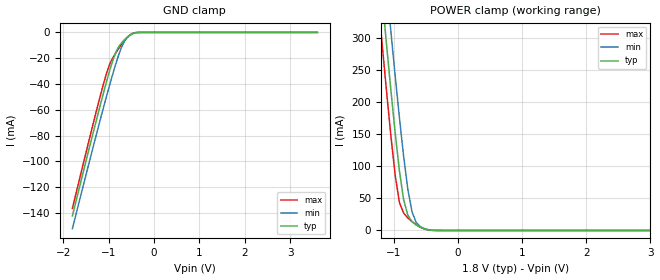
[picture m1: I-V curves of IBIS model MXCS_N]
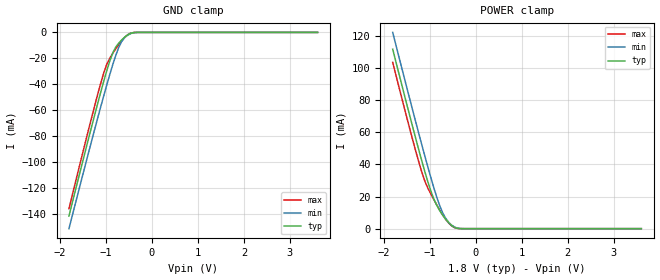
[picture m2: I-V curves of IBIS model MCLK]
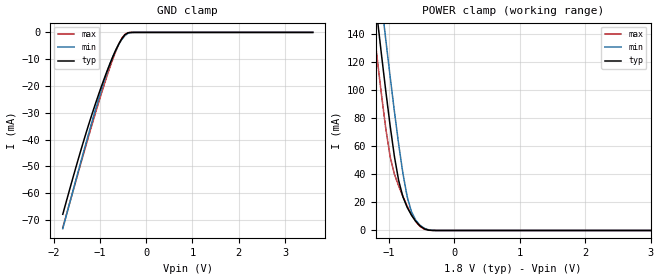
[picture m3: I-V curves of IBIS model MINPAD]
| Created by SiliconSmart  O-2018.09-SP2-3
[IBIS Ver]   4.0
[File Name]   as1101wa_rev1p4.ibs
[File Rev]   1.4
[Date]   Thursday Mar 21 2024
|[Source]   Avalanche Team
|[Notes]   Generated IBIS models from Silicon Smart
|[Rev 1.0]  Initial Release based on extracted netlist
|   Characterization
|[Rev 1.1]  Update Package RLC
|[Rev 1.2]  Recharacterize MIOPAD with Hspice run in high accuracy mode
|[Rev 1.3]  Recharacterize with Hspice to align with datasheet parameter
|[Rev 1.4]  Update the pin to the package pinout assignment
|[Disclaimer]   THE MODEL LIBRARIES ARE PROVIDED AS IS.
|[Copyright]   Copyright 2019, Avalanche Technology., All Rights Reserved
[Component]   AS10xx101_WSON
[Manufacturer] Avalanche Technology
| CONTENT :
| This file contains IBIS MODEL for PSRAM device
| AS1001101 AS1004101 AS1008101 AS1016101
| USAGE :
| The models are derived for the 1.71V to 2.0V I/O Operation.
| Temperatures for model generation: typ: 25, max: -40, min: 105
| Voltages : typ: 1.8V, min: 1.71V, max: 2.0V
| PACKAGES SUPPORTED :
| 8-pad WSON (5.0mm x 6.0mm)
| VERIFICATION :
| Errors  : 0
| Warnings: 10
| All warnings due to non-monotonic data
[Package]
|variable   typ   min   max
R_pkg   8.90E-04   8.89E-04  8.91E-04
L_pkg   1.185E-09  1.18E-09  1.19E-09
C_pkg   2.30E-13   2.21E-13  2.39E-13
[Pin]   signal_name   model_name   R_pin   L_pin   C_pin
1   CS#   MXCS_N   1.05E-01  1.35E-09  9.16E-14
2   SO   MIOPAD   1.05E-01  1.35E-09  9.16E-14
3   WP#   MINPAD   1.05E-01  1.35E-09  9.16E-14
5   SI   MINPAD   3.75E-02  3.89E-10  4.24E-14
6   CLK   MCLK   3.75E-02  3.89E-10  4.24E-14
7   HOLD#   MINPAD   3.75E-02  3.89E-10  4.24E-14
4   VSS   GND   NA   NA   NA
8   VCC   POWER   NA   NA   NA
[Model Selector] MIOPAD
| Model Description
M3_IOPAD_NVCR_OB04   45 Ohms drv strength
| Models and submodels in the file (4): MXCS_N (Input), MCLK (Input), MINPAD (Input), M3_IOPAD_NVCR_OB04 (Output)
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| XCS_N
[Model] MXCS_N
Model_type Input
Enable   Active-High
Vinl  =  0.54
Vinh  =  1.26
| Capacitance  typ   min   max
C_comp   3.084351e-12   2.813138e-12   3.400928e-12
| Variables   typ   min   max
[GND Clamp Reference]   0   0   0
[POWER Clamp Reference]   1.8   1.71   2
[Pulldown Reference]   0   0   0
[Pullup Reference]   1.8   1.71   2
[Temperature Range]   25   105   -40
[Voltage Range]   1.8   1.71   2
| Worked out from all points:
|   GND clamp passes 1 mA (typ) near -0.48 V on its own axis
|   POWER clamp passes 1 mA (typ) near -0.46 V on its own axis
[GND Clamp]
| Voltage   I(typ)   I(min)   I(max)
-1.8V     -142.2mA   -152mA     -136.3mA
-1.303V   -72.38mA   -83.46mA   -65.31mA
-1.173V   -54.66mA   -65.96mA   -47.51mA
-1.043V   -37.59mA   -48.87mA   -31.14mA
-977.6mV  -29.52mA   -40.56mA   -24.56mA
-847.2mV  -15.78mA   -24.8mA    -16.17mA
-716.9mV  -8.18mA    -11.5mA    -9.334mA
-651.7mV  -5.669mA   -6.824mA   -6.326mA
-586.6mV  -3.535mA   -3.869mA   -3.746mA
-456.2mV  -640.4uA   -879uA     -510.8uA
-325.9mV  -14.45uA   -51.53uA   -3.775uA
3.6V      0A         0A         0A
[POWER Clamp]
| Voltage   I(typ)   I(min)   I(max)
-1.8V     1.062A     1.152A     991.6mA
-1.238V   424.5mA    517.2mA    351.4mA
-1.173V   353.2mA    445.8mA    280.1mA
-1.108V   283.2mA    375.4mA    210.6mA
-1.043V   215.2mA    306.4mA    144.3mA
-977.6mV  150.6mA    239.2mA    85.02mA
-912.4mV  92.52mA    174.9mA    43.53mA
-847.2mV  47.97mA    115.2mA    27.04mA
-716.9mV  13.61mA    29.16mA    13.92mA
-651.7mV  8.604mA    12.47mA    8.943mA
-325.9mV  22.75uA    80.1uA     9.962uA
3.6V      0A         0A         0A
| CLK
[Model] MCLK
Model_type Input
Enable   Active-High
Vinl  =  0.54
Vinh  =  1.26
| Capacitance  typ   min   max
C_comp   2.700843e-12   2.498345e-12   2.928788e-12
| Variables   typ   min   max
[GND Clamp Reference]   0   0   0
[POWER Clamp Reference]   1.8   1.71   2
[Pulldown Reference]   0   0   0
[Pullup Reference]   1.8   1.71   2
[Temperature Range]   25   105   -40
[Voltage Range]   1.8   1.71   2
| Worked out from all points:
|   GND clamp passes 1 mA (typ) near -0.48 V on its own axis
|   POWER clamp passes 1 mA (typ) near -0.47 V on its own axis
[GND Clamp]
| Voltage   I(typ)   I(min)   I(max)
-1.8V     -141.2mA   -150.9mA   -135.5mA
-1.303V   -71.9mA    -82.87mA   -64.94mA
-1.173V   -54.3mA    -65.5mA    -47.25mA
-1.043V   -37.35mA   -48.53mA   -30.99mA
-977.6mV  -29.34mA   -40.29mA   -24.44mA
-847.2mV  -15.7mA    -24.65mA   -16.09mA
-716.9mV  -8.148mA   -11.44mA   -9.29mA
-651.7mV  -5.65mA    -6.8mA     -6.299mA
-586.6mV  -3.525mA   -3.859mA   -3.733mA
-456.2mV  -639.6uA   -877.8uA   -510.2uA
-325.9mV  -14.45uA   -51.53uA   -3.775uA
3.6V      0A         0A         0A
[POWER Clamp]
| Voltage   I(typ)   I(min)   I(max)
-1.8V     111.7mA    122.1mA    103.4mA
-1.369V   63.57mA    73.93mA    55.54mA
-1.238V   49.53mA    59.72mA    41.97mA
-1.108V   36.07mA    45.8mA     30.06mA
-977.6mV  23.92mA    32.38mA    21.88mA
-912.4mV  18.87mA    26mA       18.39mA
-782.1mV  11.36mA    14.53mA    11.73mA
-651.7mV  5.917mA    6.557mA    5.926mA
-521.4mV  1.955mA    2.241mA    1.736mA
-391mV    174.8uA    333.4uA    115.2uA
-260.7mV  2.189uA    12.94uA    482.3nA
3.6V      0A         0A         0A
| INPAD
[Model] MINPAD
Model_type Input
Enable   Active-High
Vinl  =  0.54
Vinh  =  1.26
| Capacitance  typ   min   max
C_comp   3.870066e-12   3.574515e-12   4.209523e-12
| Variables   typ   min   max
[GND Clamp Reference]   0   0   0
[POWER Clamp Reference]   1.8   1.71   2
[Pulldown Reference]   0   0   0
[Pullup Reference]   1.8   1.71   2
[Temperature Range]   25   105   -40
[Voltage Range]   1.8   1.71   2
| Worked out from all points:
|   GND clamp passes 1 mA (typ) near -0.46 V on its own axis
|   POWER clamp passes 1 mA (typ) near -0.44 V on its own axis
[GND Clamp]
| Voltage   I(typ)   I(min)   I(max)
-1.8V     -67.84mA   -73.19mA   -72.81mA
-1.499V   -49.26mA   -53.93mA   -54.28mA
-1.303V   -37.87mA   -41.64mA   -42.4mA
-1.108V   -27.29mA   -29.68mA   -30.84mA
-912.4mV  -17.6mA    -18.46mA   -19.84mA
-782.1mV  -11.7mA    -11.87mA   -13.01mA
-651.7mV  -6.447mA   -6.494mA   -6.896mA
-521.4mV  -2.255mA   -2.526mA   -2.141mA
-456.2mV  -849.3uA   -1.156mA   -679.4uA
-391mV    -172uA     -356.5uA   -88.88uA
-260.7mV  -2.088uA   -12.98uA   -254.3nA
3.6V      0A         0A         0A
[POWER Clamp]
| Voltage   I(typ)   I(min)   I(max)
-1.8V     419.8mA    456.6mA    390.9mA
-1.238V   178mA      215.7mA    148.4mA
-1.173V   151mA      188.6mA    121.7mA
-1.108V   124.5mA    161.8mA    96mA
-1.043V   98.85mA    135.4mA    72.14mA
-977.6mV  74.56mA    109.6mA    52.56mA
-912.4mV  52.76mA    84.78mA    40.16mA
-847.2mV  35.48mA    61.36mA    31.71mA
-716.9mV  16.42mA    23.91mA    17.31mA
-651.7mV  10.9mA     13.27mA    11.28mA
-456.2mV  1.168mA    1.554mA    921.1uA
3.6V      0A         0A         0A
